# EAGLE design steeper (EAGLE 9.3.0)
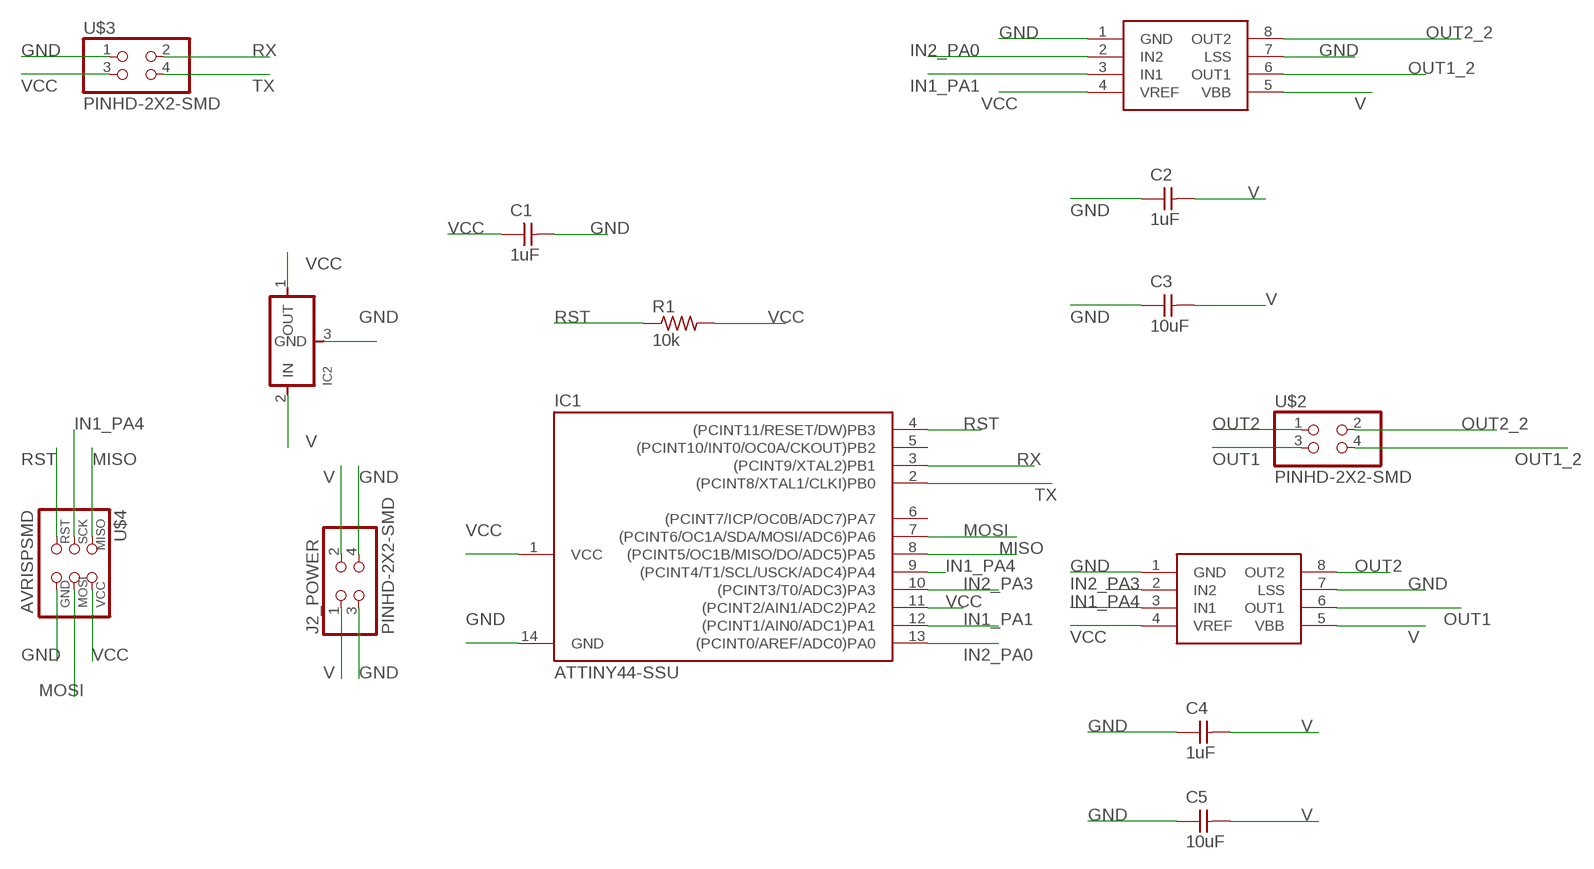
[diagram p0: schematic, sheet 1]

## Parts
C1  1uF  CAP-UNPOLARIZEDFAB  [C1206FAB]
C2  1uF  CAP-UNPOLARIZEDFAB  [C1206FAB]
C3  10uF  CAP-UNPOLARIZEDFAB  [C1206FAB]
C4  1uF  CAP-UNPOLARIZEDFAB  [C1206FAB]
C5  10uF  CAP-UNPOLARIZEDFAB  [C1206FAB]
IC1  ATTINY44-SSU  [SOIC14]
IC2  REGULATORSOT23  [SOT23]
J2_POWER  PINHD-2X2-SMD  [2X02SMD]
MOTOR1  A4953-H-BRIDGE-MOTOR-DRIVER  [SOIC8]
MOTOR2  A4953-H-BRIDGE-MOTOR-DRIVER  [SOIC8]
R1  10k  RES-US1206FAB  [R1206FAB]
U$2  PINHD-2X2-SMD  [2X02SMD]
U$3  PINHD-2X2-SMD  [2X02SMD]
U$4  AVRISPSMD  [2X03SMD]

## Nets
GND: C1.2 C2.1 C3.1 C4.1 C5.1 IC1.14(GND) IC2.3(GND) J2_POWER.3 J2_POWER.4 MOTOR1.1(GND) MOTOR1.7(LSS) MOTOR2.1(GND) MOTOR2.7(LSS) U$3.1 U$4.6(GND)
IN1_PA1: IC1.12((PCINT1/AIN0/ADC1)PA1) MOTOR2.3(IN1)
IN1_PA4: IC1.9((PCINT4/T1/SCL/USCK/ADC4)PA4) MOTOR1.3(IN1) U$4.3(SCK)
IN2_PA0: IC1.13((PCINT0/AREF/ADC0)PA0) MOTOR2.2(IN2)
IN2_PA3: IC1.10((PCINT3/T0/ADC3)PA3) MOTOR1.2(IN2)
MISO: IC1.8((PCINT5/OC1B/MISO/DO/ADC5)PA5) U$4.1(MISO)
MOSI: IC1.7((PCINT6/OC1A/SDA/MOSI/ADC6)PA6) U$4.4(MOSI)
OUT1: MOTOR1.6(OUT1) U$2.3
OUT1_2: MOTOR2.6(OUT1) U$2.4
OUT2: MOTOR1.8(OUT2) U$2.1
OUT2_2: MOTOR2.8(OUT2) U$2.2
RST: IC1.4((PCINT11/RESET/DW)PB3) R1.1 U$4.5(RST)
RX: IC1.3((PCINT9/XTAL2)PB1) U$3.2
TX: IC1.2((PCINT8/XTAL1/CLKI)PB0) U$3.4
V: C2.2 C3.2 C4.2 C5.2 IC2.2(IN) J2_POWER.1 J2_POWER.2 MOTOR1.5(VBB) MOTOR2.5(VBB)
VCC: C1.1 IC1.1(VCC) IC1.11((PCINT2/AIN1/ADC2)PA2) IC2.1(OUT) MOTOR1.4(VREF) MOTOR2.4(VREF) R1.2 U$3.3 U$4.2(VCC)
Unconnected: IC1.5((PCINT10/INT0/OC0A/CKOUT)PB2) IC1.6((PCINT7/ICP/OC0B/ADC7)PA7)

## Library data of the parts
C1-C5 = eagle_fab:CAP-UNPOLARIZED
IC1 = eagle_fab:ATTINY44
IC2 = eagle_fab:REGULATOR
J2_POWER U$2 U$3 = eagle_fab:PINHD-2X2-SMD
MOTOR1 MOTOR2 = eagle_fab:A4953-H-BRIDGE-MOTOR-DRIVER
R1 = eagle_fab:RES-US: Resistor (US Symbol)
U$4 = eagle_fab:AVRISP

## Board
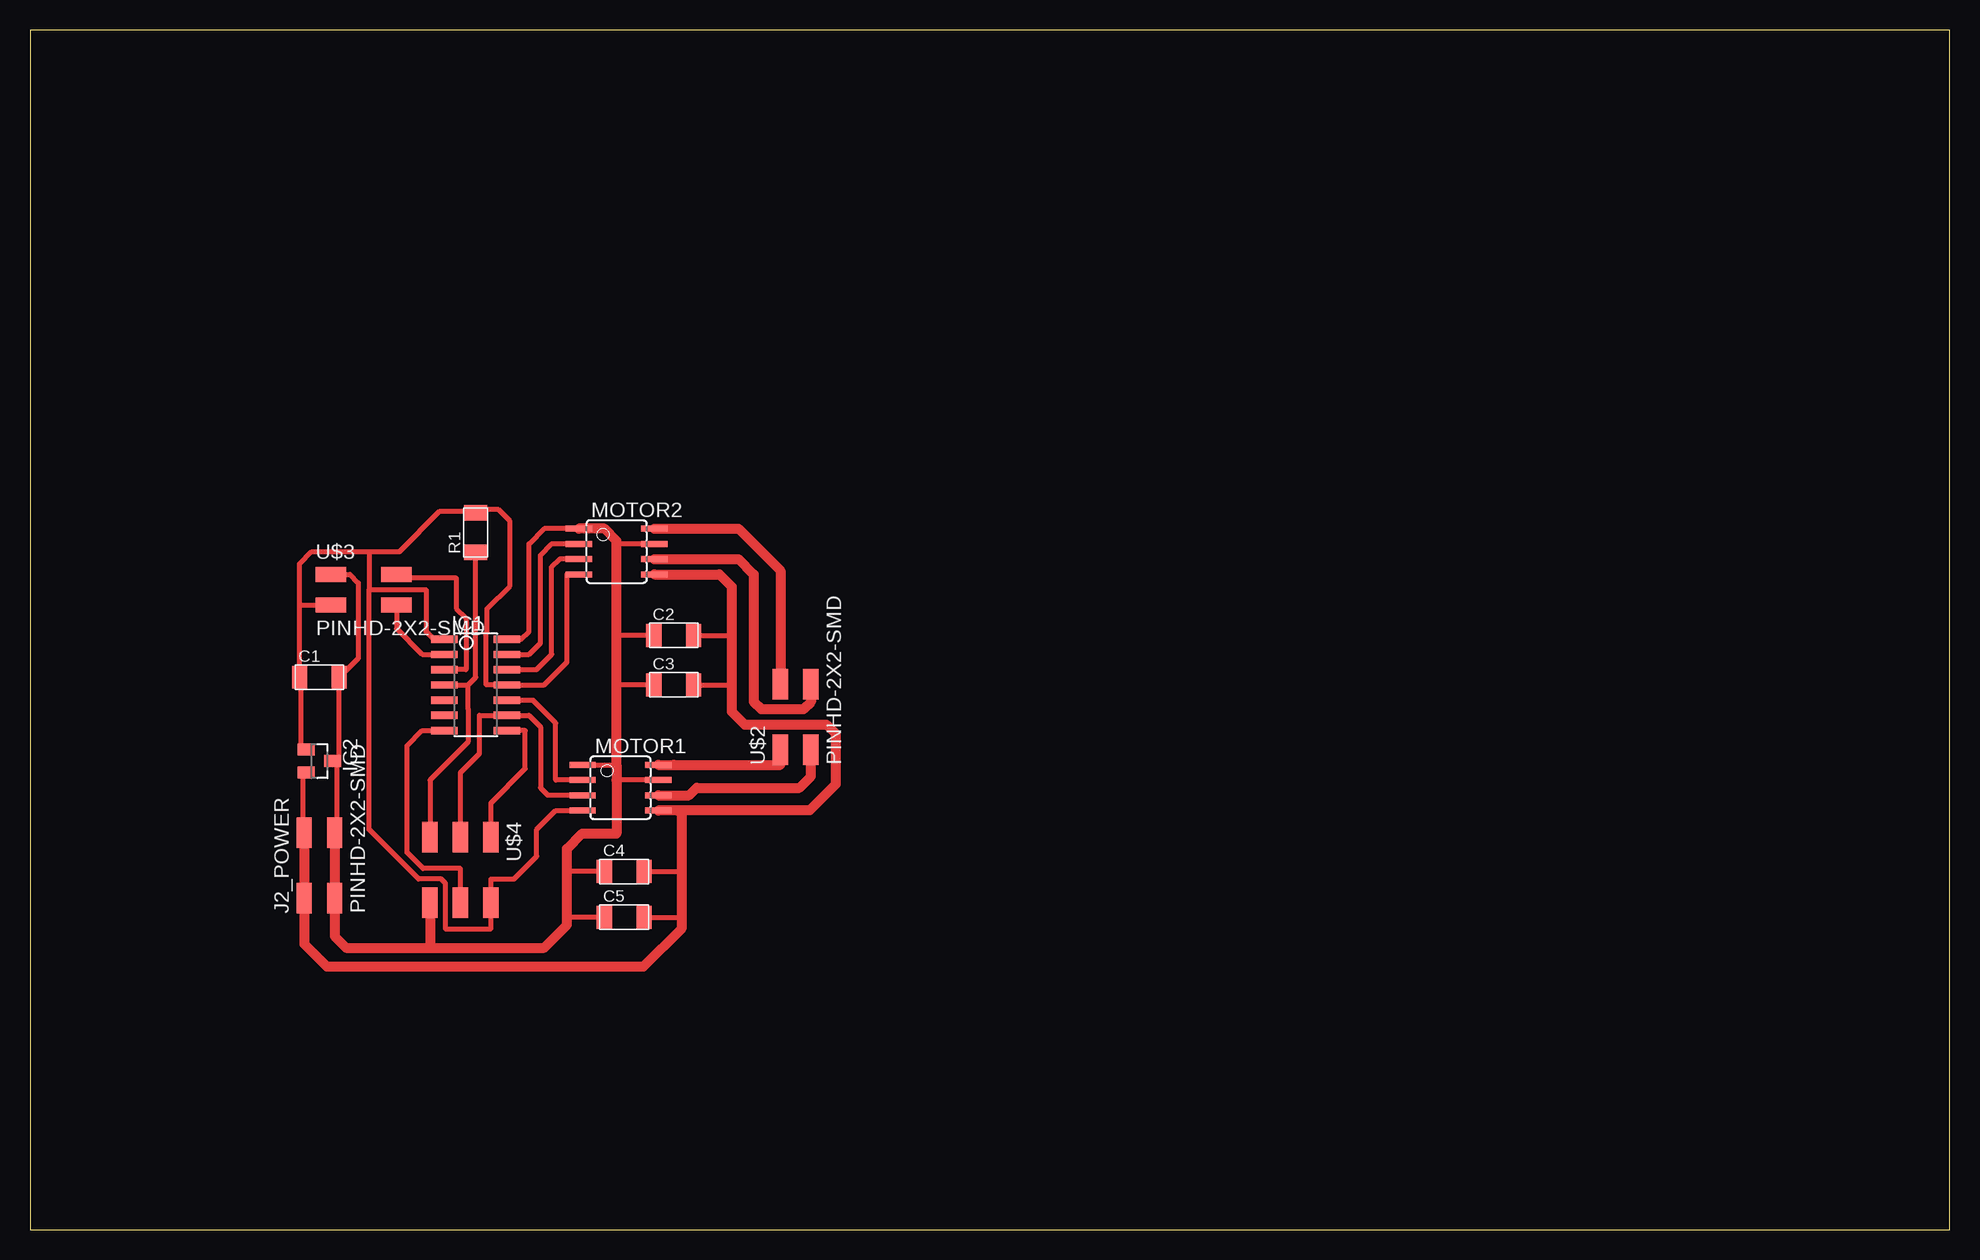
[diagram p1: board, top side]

Size 160 x 100 mm. Coordinates in mm from the lower left corner, seen from the top.
Outline: 0,0 160,0 160,100 0,100 0,0
Copper layers (1*16): Top 0.035mm / dielectric 1.5mm / Bottom 0.035mm
Design rules "eagle_fabcity-designrules *": minimum track width 16mil, minimum drill 32mil, track to track 16mil, track to pad 16mil, pad to pad 16mil, via to via 16mil, smd to smd 16mil, copper to edge 16mil, drill to drill 16mil, minimum pad ring 10mil, minimum via ring 8mil, stop-mask expansion 4mil, vias tented up to drill 0mil, thermal gap 16mil

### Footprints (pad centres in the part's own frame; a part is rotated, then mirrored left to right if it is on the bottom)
C1206FAB = smd 1.27 x 1.905: 1 -1.651,0; 2 1.651,0
SOIC14 = smd 0.61 x 2.21: 1 -3.81,-2.603; 2 -2.54,-2.603; 3 -1.27,-2.603; 4 0,-2.603; 5 1.27,-2.603; 6 2.54,-2.603; 7 3.81,-2.603; 8 3.81,2.603; 9 2.54,2.603; 10 1.27,2.603; 11 0,2.603; 12 -1.27,2.603; 13 -2.54,2.603; 14 -3.81,2.603
SOT23 = smd 1 x 1.4: 1 -0.95,-1.1; 2 0.95,-1.1; 3 0,1.1
2X02SMD = smd 2.54 x 1.27: 1 -2.54,1.27; 2 2.92,1.27; 3 -2.54,-1.27; 4 2.92,-1.27
SOIC8 = smd 0.5 x 2.2: 1 -1.905,-3.154; 2 -0.645,-3.154; 3 0.625,-3.154; 4 1.895,-3.154; 5 1.905,3.154; 6 0.635,3.154; 7 -0.635,3.154; 8 -1.905,3.154
R1206FAB = smd 1.27 x 1.905: 1 -1.651,0; 2 1.651,0
2X03SMD = smd 2.54 x 1.27: 1 -2.54,2.54; 2 2.92,2.54; 3 -2.54,0; 4 2.92,0; 5 -2.54,-2.54; 6 2.92,-2.54

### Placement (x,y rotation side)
C1  24.13,46.04 0 top
C2  53.66,49.53 0 top
C3  53.66,45.4 0 top
C4  49.53,29.84 0 top
C5  49.53,26.04 0 top
IC1  37.15,45.4 270 top
IC2  24.13,39.05 270 top
J2_POWER  24.13,30.16 90 top
MOTOR1  49.21,36.83 270 top
MOTOR2  48.9,56.52 270 top
R1  37.15,58.1 90 top
U$2  63.82,42.55 90 top
U$3  27.62,53.34 0 top
U$4  35.88,30.16 270 top

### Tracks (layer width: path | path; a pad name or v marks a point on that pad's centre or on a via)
GND
  Top 0.406: IC2.3 25.55,38.73 | 25.55,38.73 25.55,33.23 J2_POWER.4 | 25.55,38.73 25.72,38.91 25.72,45.97 C1.2 27.37,47.62 27.37,53.91 26.67,54.61 U$3.1 | IC1.14 40.96,49.21 41.59,49.85 41.59,57.15 42.86,58.42 MOTOR2.1 | MOTOR1.1 48.9,38.73 | MOTOR1.7 48.9,37.47 | C4.1 44.77,29.84 | C5.1 44.77,26.04 | MOTOR2.7 49.15,57.15 48.9,57.4 | C3.1 48.9,45.4 | C2.1 48.9,49.53
  Top 0.813: J2_POWER.4 J2_POWER.3 25.4,24.45 26.35,23.5 33.34,23.5 | 33.34,23.5 42.86,23.5 44.77,25.4 44.77,26.04 44.77,29.84 44.77,31.75 46.04,33.02 48.9,33.02 48.9,37.47 48.9,38.73 48.9,45.4 48.9,49.53 48.9,57.4 47.88,58.42 MOTOR2.1 | U$4.6 33.34,23.5
IN1_PA1
  Top 0.406: MOTOR2.3 44.13,55.89 43.5,55.26 43.5,47.94 42.23,46.67 IC1.12
IN1_PA4
  Top 0.406: MOTOR1.3 44.15,36.2 44.14,36.2 43.18,36.2 42.55,36.83 42.55,41.91 41.59,42.86 IC1.9 37.47,42.86 37.47,39.69 35.88,38.1 U$4.3
IN2_PA0
  Top 0.406: IC1.13 41.59,47.94 42.55,48.9 42.55,56.21 43.5,57.16 MOTOR2.2
IN2_PA3
  Top 0.406: IC1.10 41.91,44.13 43.81,42.23 43.81,37.48 MOTOR1.2
MISO
  Top 0.406: U$4.1 38.42,35.56 41.27,38.42 41.27,41.59 IC1.8
MOSI
  Top 0.406: U$4.4 35.88,30.1 32.77,30.1 31.43,31.43 31.43,40.32 32.7,41.59 IC1.7
OUT1
  Top 0.813: MOTOR1.6 54.93,36.2 55.56,36.83 64.14,36.83 65.09,37.78 U$2.3
OUT1_2
  Top 0.813: MOTOR2.6 59.05,55.88 60.33,54.61 60.33,44 60.94,43.38 64.47,43.38 65.09,44 U$2.4
OUT2
  Top 0.813: 53.66,38.73 MOTOR1.8 62.55,38.73 U$2.1
OUT2_2
  Top 0.813: MOTOR2.8 59.05,58.42 62.55,54.93 U$2.2
RST
  Top 0.406: U$4.5 33.34,37.47 36.51,40.64 36.51,43.43 36.51,45.4 | IC1.4 36.51,45.4 | R1.1 37.15,46.04 36.51,45.4
RX
  Top 0.406: U$3.2 30.86,54.29 35.52,54.29 35.52,51.78 36.34,50.96 36.34,46.67 IC1.3
TX
  Top 0.406: U$3.4 30.54,50.1 32.7,47.94 IC1.2
V
  Top 0.406: IC2.2 22.71,37.78 22.71,33.23 J2_POWER.2 | C5.2 54.29,26.04 | C4.2 54.29,29.84 | C2.2 58.48,49.53 | C3.2 58.48,45.4
  Top 0.813: J2_POWER.2 J2_POWER.1 22.86,23.81 24.77,21.91 51.12,21.91 54.29,25.08 54.29,26.04 54.29,29.84 54.29,34.92 53.98,34.92 | 53.98,34.92 MOTOR1.5 | MOTOR2.5 57.47,54.61 58.48,53.59 58.48,49.53 58.48,45.4 58.48,43.18 59.58,42.09 66.38,42.09 67.17,41.29 67.17,37.13 65.02,34.98 54.03,34.98 53.98,34.92
VCC
  Top 0.406: 28.26,56.52 28.26,53.34 | 28.26,56.52 23.5,56.52 22.48,55.5 22.48,52.07 | 28.26,53.34 33.02,53.34 33.02,49.85 33.66,49.21 IC1.1 | MOTOR2.4 44.77,54.62 44.77,47.31 42.86,45.4 IC1.11 38.04,45.4 38.04,49.77 38.1,49.83 38.1,51.75 40.01,53.66 40.01,59.05 39.05,60.01 37.4,60.01 37.27,59.88 | 28.26,53.34 28.26,33.34 32.38,29.21 34.29,29.21 34.61,28.89 34.61,25.08 38.42,25.08 U$4.2 38.42,29.21 40.33,29.21 42.23,31.11 42.23,33.34 43.81,34.92 46.05,34.92 MOTOR1.4 | 37.27,59.88 R1.2 | 28.26,56.52 30.8,56.52 34.16,59.88 37.27,59.88 | IC2.1 22.54,40 22.54,45.97 C1.1 22.48,52.07 | 22.48,52.07 U$3.3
